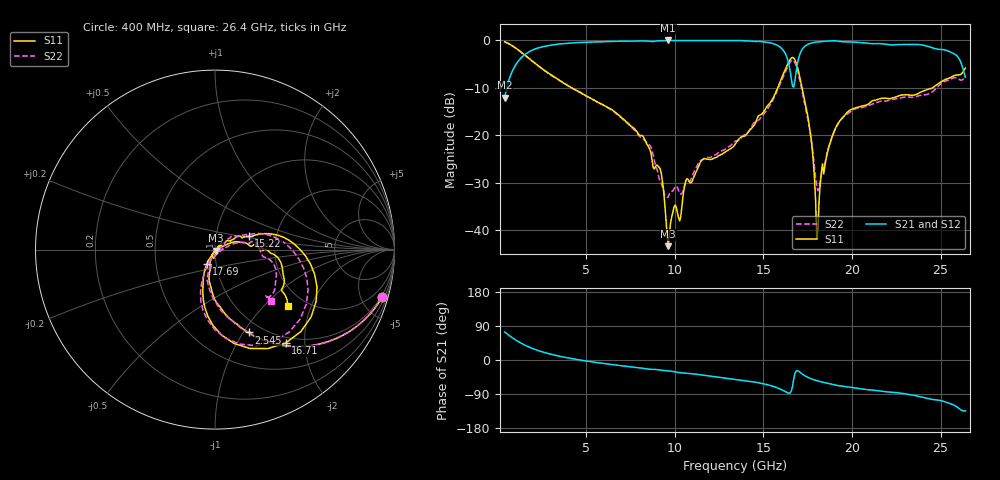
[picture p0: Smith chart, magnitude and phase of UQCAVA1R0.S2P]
!  Part Number  UQCAVA1R0 	Mounting Orientation: Horizontal
!  Description: Ultra Low ESR Microwave capacitors
!  Application: Coupling, Bypass, Tuning, DC Block
!  Filters, Matching
# GHZ S DB R 50
! Freq  |S11|  S11 Ph  |S21|  S21 Ph  |S12|  S12 Ph  |S22|  S22 Ph
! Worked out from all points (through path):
!   401 points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, 400 MHz to 26.4 GHz, reference 50 ohm
!   highest |S21| = 0.00 dB at 9.63 GHz (marker M1); lowest = -12.1 dB at 400 MHz (marker M2)
!   group delay of S21, straight-line fit = 15.5 ps
!   lowest |S11| = -43.4 dB at 9.63 GHz (marker M3), VSWR 1.01, Z = 50.3 - j0.59 ohm
!   |S11| at or under -10 dB: 4.2 GHz to 15.81 GHz (11.61 GHz wide, 116 % of centre); 17.18 GHz to 24.54 GHz (7.357 GHz wide, 35.3 % of centre)
!   |S22| runs from -33.1 to -0.3 dB; largest |S21 - S12| = 0.0044
!   S11 on the Smith chart (normalised r, x): 400 MHz: 0.85, -7.16; 2.545 GHz: 0.86, -1.06; 15.22 GHz: 1.44, +0.22; 16.71 GHz: 0.90, -1.63; 17.69 GHz: 0.90, -0.15; 26.4 GHz: 1.64, -1.38
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0.4  -0.28 -15.7  -12.08 74.1  -12.08 74.1  -0.29 -15.8
1.245  -2.21 -43.1  -4.03 46.6  -4.04 46.5  -2.23 -43.2
2.545  -6.05 -67.8  -1.34 21.2  -1.34 21.1  -6.08 -68.4
4.755  -11.15 -90.6  -0.41 -0.8  -0.41 -0.9  -11.24 -91.8
8.525  -22.48 -110.8  -0.13 -23.9  -0.12 -23.9  -21.87 -105.7
9.11  -26.73 -101.9  -0.06 -26.0  -0.05 -26.0  -28.98 -103.9
9.63  -43.41 -60.2  0.00 -28.6  -0.01 -28.6  -33.05 -53.8
11.515  -25.30 41.8  -0.01 -39.5  -0.01 -39.5  -25.25 27.0
13.4  -21.95 36.5  -0.01 -51.2  -0.01 -51.3  -21.30 38.7
15.22  -13.87 21.6  -0.39 -65.1  -0.38 -65.2  -14.50 26.3
16.13  -7.05 3.9  -2.12 -80.6  -2.11 -80.7  -7.61 1.7
16.715  -3.71 -52.8  -9.82 -50.2  -9.81 -50.3  -4.32 -57.4
17.105  -8.62 -96.3  -2.47 -33.6  -2.45 -33.8  -9.27 -101.2
17.69  -20.60 -119.3  -0.56 -49.5  -0.55 -49.6  -20.57 -115.4
17.755  -22.80 -121.0  -0.50 -50.6  -0.49 -50.7  -22.35 -113.8
17.95  -33.96 -112.1  -0.37 -53.7  -0.35 -53.8  -28.99 -92.2
18.08  -40.11 9.9  -0.31 -55.4  -0.30 -55.6  -31.75 -53.2
18.34  -26.04 43.1  -0.22 -58.4  -0.22 -58.5  -27.01 4.5
19.25  -17.28 18.2  -0.18 -67.9  -0.17 -68.0  -17.43 16.5
22.11  -12.27 1.2  -0.88 -84.8  -0.87 -84.9  -12.60 9.1
25.23  -8.31 -13.9  -1.99 -110.0  -1.99 -110.2  -8.64 -22.3
26.4  -5.83 -37.6  -7.76 -134.0  -7.75 -134.2  -7.40 -42.6
